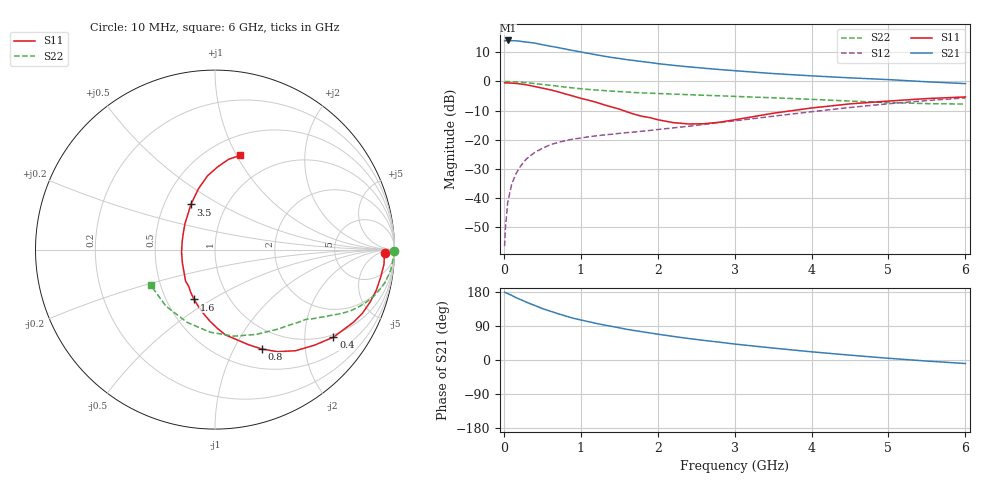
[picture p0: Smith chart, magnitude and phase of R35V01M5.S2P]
! SIEMENS Small Signal Semiconductors
! BFR181
! Si NPN RF Bipolar Junction Transistor in SOT23
! VCE = 5 V  IC = 1.5 mA
! Common Emitter S-Parameters:  May  1996
# GHz  S  MA  R  50
!  f  S11  S21  S12  S22
! GHz  MAG  ANG  MAG  ANG  MAG  ANG  MAG  ANG
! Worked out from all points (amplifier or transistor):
!   36 points, 10 MHz to 6 GHz, reference 50 ohm
!   highest |S21| = 14.1 dB at 50 MHz (marker M1)
!   |S21| within 3 dB of that: start of sweep to 813.1 MHz
!   unconditionally stable (mu >= 1): 1.774 GHz to 3.537 GHz
!   at 250 MHz: K = 0.19, MSG = 20.8 dB, |S12| = -27.9 dB
!   at 1.4 GHz: K = 0.87, MSG = 13.2 dB, |S12| = -18.1 dB
!   at 6 GHz: K = 0.86, MSG = 2.5 dB, |S12| = -5.6 dB
!   S11 on the Smith chart (normalised r, x): 10 MHz: 34, -11; 400 MHz: 0.92, -2.76; 800 MHz: 0.73, -1.29; 1.6 GHz: 0.69, -0.42; 3.5 GHz: 0.68, +0.37; 6 GHz: 0.69, +1.03
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0.01  0.9478 -1.0  4.974 179.2  0.0015 98.4  0.9983 -0.4
0.02  0.9441 -2.0  4.972 177.9  0.003 86.0  0.9958 -1.0
0.05  0.9452 -4.9  5.047 175.3  0.0084 88.2  0.9962 -2.3
0.1  0.9362 -9.3  4.98 171.0  0.0169 84.8  0.9903 -4.4
0.15  0.9265 -14.3  4.98 165.3  0.025 80.3  0.9853 -6.7
0.2  0.9123 -18.7  4.932 161.0  0.0328 78.3  0.9748 -8.8
0.3  0.8724 -27.5  4.718 152.0  0.0478 73.1  0.9521 -12.7
0.4  0.8206 -36.5  4.558 144.1  0.0606 68.2  0.9224 -16.3
0.5  0.7685 -43.9  4.265 135.8  0.0714 64.4  0.8897 -19.4
0.6  0.7206 -51.4  4.026 129.1  0.0819 60.7  0.8596 -21.9
0.8  0.6109 -64.9  3.601 116.2  0.0967 55.4  0.8013 -26.0
0.9  0.5626 -70.5  3.393 110.4  0.1029 53.6  0.7736 -27.7
1.1  0.4781 -83.1  3.033 101.1  0.1125 51.4  0.7295 -30.5
1.3  0.3995 -94.1  2.717 92.6  0.121 50.0  0.698 -32.7
1.6  0.3015 -112.8  2.363 80.9  0.1327 49.6  0.6608 -35.8
1.9  0.2397 -133.3  2.111 71.3  0.1448 51.0  0.6289 -38.9
2.2  0.197 -157.1  1.892 62.3  0.1598 52.0  0.6077 -42.5
3  0.22 139.8  1.53 42.1  0.2113 53.7  0.555 -54.0
3.5  0.2851 118.1  1.366 31.5  0.2535 52.8  0.5249 -64.3
4.5  0.4129 95.8  1.153 12.8  0.358 46.1  0.461 -93.4
5.5  0.509 81.4  0.987 -2.8  0.4704 33.9  0.4171 -131.0
6  0.5428 75.1  0.919 -9.3  0.5224 26.4  0.4095 -151.3
